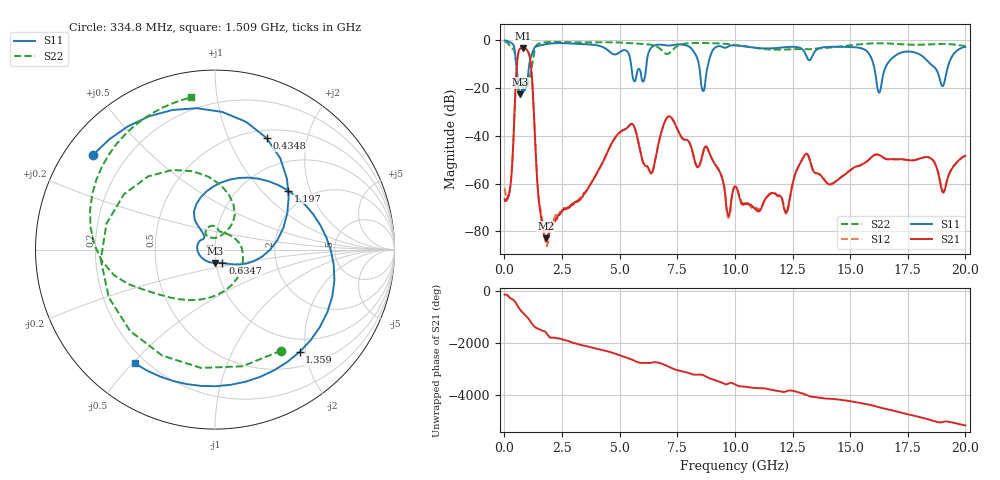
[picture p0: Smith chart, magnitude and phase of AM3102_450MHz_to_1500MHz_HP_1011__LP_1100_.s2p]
!Agilent Technologies,E8364B,MY43040894,A.07.50.67
!Agilent E8364B: A.07.50.67
!Date: Thursday, January 11, 2018 06:26:07
!Correction: S11(Full 2 Port(1,2))
!S21(Full 2 Port(1,2))
!S12(Full 2 Port(1,2))
!S22(Full 2 Port(1,2))
!S2P File: Measurements: S11, S21, S12, S22:
# Hz S  dB  R 50
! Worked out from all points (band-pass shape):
!   1601 points, 10 MHz to 20 GHz, reference 50 ohm
!   highest |S21| = -3.17 dB at 797.1 MHz (marker M1); lowest = -83.0 dB at 1.797 GHz (marker M2)
!   |S21| within 3 dB of the highest: 589.7 MHz to 1.084 GHz (494.4 MHz wide, 59.1 % of centre)
!   lowest |S11| = -22.5 dB at 684.7 MHz (marker M3), VSWR 1.16, Z = 49.4 - j7.44 ohm
!   |S11| at or under -10 dB: 5.495 GHz to 6.164 GHz (668.7 MHz wide, 11.5 % of centre); 16.01 GHz to 16.6 GHz (593.2 MHz wide, 3.64 % of centre); 18.5 GHz to 19.27 GHz (774.8 MHz wide, 4.1 % of centre)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
!   |S22| runs from -23.7 to -0.5 dB; largest |S21 - S12| = 0.0011
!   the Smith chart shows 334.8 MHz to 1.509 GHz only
!   S11 on the Smith chart (normalised r, x): 334.8 MHz: 0.08, +0.34; 434.8 MHz: 0.59, +1.39; 634.7 MHz: 1.07, -0.16; 1.197 GHz: 1.58, +1.43; 1.359 GHz: 0.75, -1.89; 1.509 GHz: 0.16, -0.51
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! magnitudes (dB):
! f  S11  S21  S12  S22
! 10 MHz  0.0  -66.5  -62.0  -0.5
! 334.8 MHz  -1.3  -52.7  -52.2  -3.4
! 434.8 MHz  -3.3  -31.5  -31.3  -4.5
! 634.7 MHz  -21.5  -4.2  -4.2  -23.1
! 684.7 MHz  -22.5  -3.5  -3.5  -23.5
! 797.1 MHz  -19.9  -3.2  -3.2  -17.8
! 1.197 GHz  -5.6  -15.8  -15.8  -10.7
! 1.359 GHz  -2.6  -47.5  -47.3  -2.5
! 1.509 GHz  -2.2  -68.3  -67.3  -1.3
! 1.797 GHz  -1.6  -83.0  -84.3  -0.8
! 3.346 GHz  -1.6  -65.9  -65.2  -0.9
! 5.445 GHz  -7.2  -35.3  -35.4  -1.2
! 6.332 GHz  -3.5  -55.5  -55.3  -1.8
! 6.682 GHz  -1.8  -43.4  -43.4  -3.0
! 8.618 GHz  -21.2  -47.0  -46.9  -1.1
! 9.705 GHz  -2.6  -73.1  -74.1  -1.6
! 10.01 GHz  -2.1  -61.2  -61.0  -1.9
! 12.23 GHz  -2.8  -72.2  -72.7  -3.8
! 13.34 GHz  -6.9  -53.2  -53.2  -3.6
! 16.68 GHz  -9.0  -49.8  -49.8  -1.3
! 19.05 GHz  -18.7  -63.7  -63.3  -1.5
! 20 GHz  -2.7  -48.4  -48.4  -2.4
